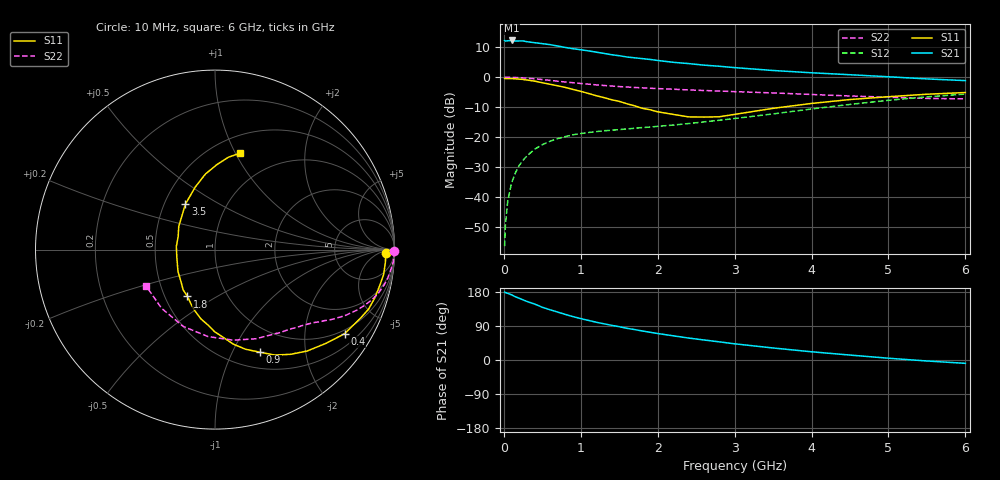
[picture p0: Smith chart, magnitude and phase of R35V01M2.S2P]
! SIEMENS Small Signal Semiconductors
! BFR181
! Si NPN RF Bipolar Junction Transistor in SOT23
! VCE = 5 V  IC = 1.2 mA
! Common Emitter S-Parameters:  May  1996
# GHz  S  MA  R  50
!  f  S11  S21  S12  S22
! GHz  MAG  ANG  MAG  ANG  MAG  ANG  MAG  ANG
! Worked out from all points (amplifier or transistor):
!   36 points, 10 MHz to 6 GHz, reference 50 ohm
!   highest |S21| = 12.3 dB at 100 MHz (marker M1)
!   |S21| within 3 dB of that: start of sweep to 967.9 MHz
!   unconditionally stable (mu >= 1): 1.945 GHz to 3.612 GHz
!   at 250 MHz: K = 0.17, MSG = 19.9 dB, |S12| = -27.7 dB
!   at 1.4 GHz: K = 0.82, MSG = 12.6 dB, |S12| = -17.7 dB
!   at 6 GHz: K = 0.86, MSG = 2.3 dB, |S12| = -5.6 dB
!   S11 on the Smith chart (normalised r, x): 10 MHz: 38, -14; 400 MHz: 0.87, -3.16; 900 MHz: 0.69, -1.29; 1.8 GHz: 0.65, -0.37; 3.5 GHz: 0.64, +0.36; 6 GHz: 0.67, +1.04
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0.01  0.9545 -1.0  4.116 179.3  0.0015 86.0  0.9989 -0.4
0.02  0.9514 -1.6  4.027 178.1  0.0033 82.6  0.998 -0.9
0.05  0.9521 -4.3  4.06 175.9  0.0084 86.4  0.9965 -2.0
0.1  0.9497 -8.4  4.118 172.0  0.017 84.7  0.9954 -4.0
0.15  0.9395 -12.3  4.026 166.9  0.0252 81.5  0.988 -6.0
0.25  0.9177 -21.2  4.041 158.6  0.041 76.1  0.9739 -9.8
0.4  0.8608 -33.0  3.78 147.6  0.0626 69.4  0.9419 -15.0
0.5  0.8087 -40.3  3.645 139.2  0.0746 65.6  0.9152 -18.0
0.6  0.763 -47.8  3.509 132.6  0.085 61.3  0.8855 -20.8
0.8  0.6756 -60.4  3.147 120.2  0.1019 55.5  0.8313 -25.3
0.9  0.6248 -66.3  2.996 114.5  0.1092 53.2  0.8104 -27.1
1.1  0.536 -79.1  2.758 104.5  0.119 50.1  0.7658 -30.3
1.2  0.4914 -84.6  2.627 99.7  0.1233 48.8  0.7452 -31.8
1.4  0.4209 -95.5  2.376 91.5  0.13 47.3  0.7123 -34.3
1.6  0.3604 -108.0  2.179 83.6  0.1369 46.8  0.6858 -36.3
1.8  0.3026 -120.5  2.046 76.6  0.1442 46.9  0.665 -38.5
2.2  0.2395 -149.4  1.777 63.9  0.1586 48.5  0.6304 -43.3
2.8  0.2182 159.9  1.526 47.9  0.1909 51.6  0.5884 -51.7
3.5  0.3021 123.1  1.296 31.7  0.2439 52.2  0.5469 -65.3
4.5  0.424 97.3  1.101 13.0  0.3515 46.8  0.4861 -94.6
5.5  0.5198 81.8  0.937 -2.6  0.4698 34.6  0.4424 -132.2
6  0.5549 75.5  0.878 -8.8  0.5229 26.9  0.4344 -152.5
